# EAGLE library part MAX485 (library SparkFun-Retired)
RS-485 transceiver
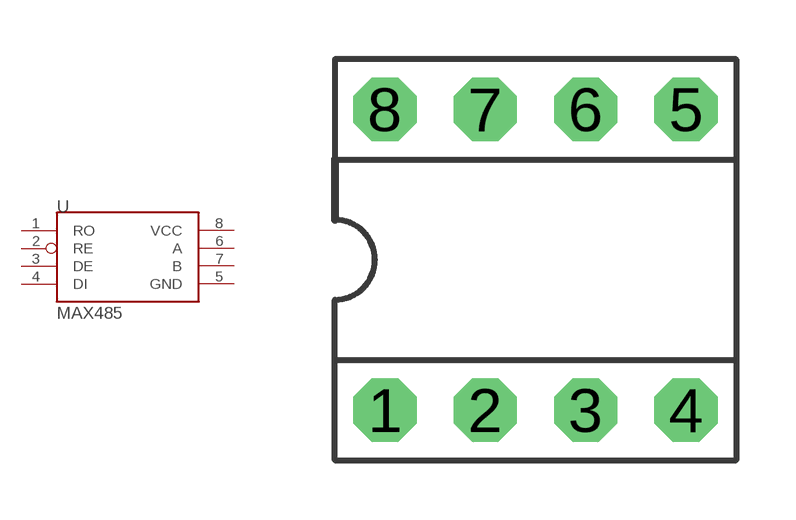
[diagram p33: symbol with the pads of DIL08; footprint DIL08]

Designator prefix -

## MAX485DIL  [DIL08]
1  RO
2  RE
3  DE
4  DI
5  GND
6  A
7  B
8  VCC

## Footprint DIL08 (pad centres in mm)
Dual In Line
drill 0.813 pad 1.6 octagon: 1 -3.81,-3.81; 2 -1.27,-3.81; 3 1.27,-3.81; 4 3.81,-3.81; 5 3.81,3.81; 6 1.27,3.81; 7 -1.27,3.81; 8 -3.81,3.81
